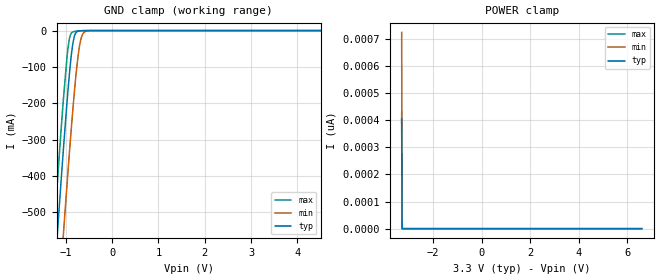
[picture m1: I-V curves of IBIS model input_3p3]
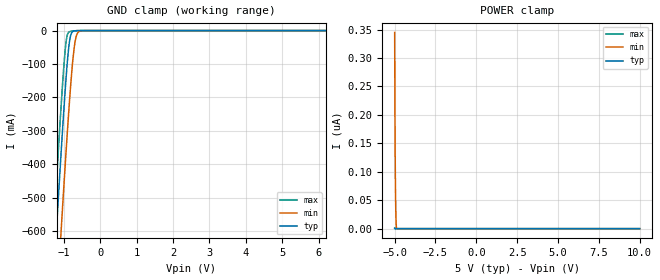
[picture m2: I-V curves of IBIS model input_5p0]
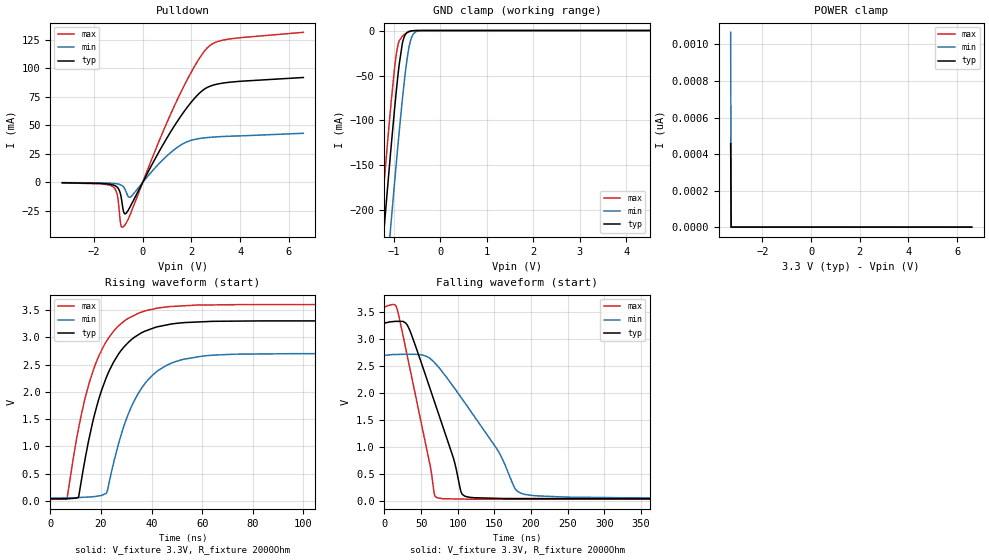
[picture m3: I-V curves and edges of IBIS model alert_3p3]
| Texas Instruments Incorporated
| INA233 High-Side or Low-Side Measurement,
| Bi-Directional Current and Power Monitor with I2C/SMBus/PMBus Compatible Interface
| Marketing part#   Digital Voltage Range   Package-type   #pins
| INA233   2.7V - 5.5V   DGS   10
[IBIS Ver]   4.1
[File name]   ina233.ibs
[Date]   04/25/2017
[File Rev]   1.0
[Source]
| Texas Instruments Incorporated.
| Analog-elab Design Center, HPA
| 12500 TI Blvd
| Dallas, TX -75243
| e-mail: elab_scm_ibis@list.ti.com
[Notes]   Revision History:
| Rev 1.0: 04/25/2017
| - Initial version of the model
| - SDA pin IBIS modeling is done for both
| - Model generated from simulations in SPECTRE
| - Model matched to SPICE simulation
| - C_comp although listed in numerical order of value are
|   obtained from varying PVT conditions. For PVT conditions for
|   each specific value refer the buffer description under
|   respective [Model]. IBIS model user is responsible for using
|   appropriate C_comp to simulate for Signal Integrity.
[Disclaimer]
| This model is designed as an aid for customers of Texas Instruments.
| TI and its licensors and suppliers make no warranties, either expressed
| or implied, with respect to this  model, including the warranties of
| merchantability or fitness for a particular purpose. The model is
| provided solely on an "as is" basis. The entire risk as to its quality
| and performance is with the customer.
[Copyright]
| (C) Copyright 2017 Texas Instruments Incorporated. All rights reserved.
|   INA233
[Component]   INA233
[Manufacturer]  TI
[Package]   |10 VSSOP   -  DGS package
|   typ   min   max
R_pkg   0   0   0
L_pkg   0   0   0
C_pkg   0   0   0
[Pin]  signal_name model_name   R_pin   L_pin   C_pin
1   A1   input   0.05873  1.44199nH  0.22518pF
2   A0   input   0.05490  1.37094nH  0.25227pF
3   Alert   alert   0.05487  1.36860nH  0.25269pF
4   SDA   sda   0.05819  1.42119nH  0.25533pF
5   SCL   scl   0.05921  1.44928nH  0.22479pF
6   VS   power   0.07038  1.61690nH  0.23536pF
7   GND   gnd   0.06315  1.49060nH  0.26023pF
8   VBUS   nc   0.06204  1.47113nH  0.26021pF
9   IN-   nc   0.05785  1.40761nH  0.25629pF
10   IN+   nc   0.07411  1.67461nH  0.23869pF
|   Model Selectors
[Model Selector] input
input_3p3   3.3V  digital Input
input_5p0   5.0V  digital Input
[Model Selector] scl
scl_3p3   3.3V  digital Input
scl_5p0   5.0V  digital Input
[Model Selector] alert
alert_3p3   3.3V  digital Open_drain
alert_5p0   5.0V  digital Open_drain
[Model Selector] sda
sda_3p3   3.3V  digital I/O_Open_drain
sda_5p0   5.0V  digital I/O_Open_drain
sda_hs_3p3   3.3V  digital I/O_Open_drain
sda_hs_5p0   5.0V  digital I/O_Open_drain
| Models and submodels in the file (10): input_3p3 (Input), input_5p0 (Input), alert_3p3 (Open_drain), alert_5p0 (Open_drain), scl_3p3 (Input), scl_5p0 (Input), sda_hs_3p3 (I/O_open_drain), sda_hs_5p0 (I/O_open_drain), sda_3p3 (I/O_open_drain), sda_5p0 (I/O_open_drain)
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|   input_3p3
[Model]   input_3p3
Model_type   Input
Vinl = 0.4
Vinh = 2.31
|   typ   min   max
C_comp   6.158E-13   5.919E-13   6.357E-13
| Where Nom  PVT is Nominal Process, 3.3V, 25C
|   Fast PVT is Strong Process,  3.6V, -40C
|   Slow PVT is Weak Process,   2.7V, 125C
[Voltage Range]   3.3   2.7   3.6
[Temperature Range]   25   125   -40
[Power Clamp Reference]   3.3   2.7   3.6
[GND Clamp Reference]   0   0   0
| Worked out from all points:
|   GND clamp passes 1 mA (typ) near -0.71 V on its own axis
[GND Clamp]
|   Voltage   I(typ)   I(min)   I(max)
-3.3V     -4.686A    -4.907A    -4.556A
-1.251V   -685.9mA   -923.4mA   -543.4mA
-1.181V   -558mA     -795.1mA   -415.7mA
-1.053V   -328.1mA   -561.6mA   -190.2mA
-953.7mV  -165.6mA   -388.9mA   -49.35mA
-904.2mV  -95.52mA   -306.4mA   -13.32mA
-844.8mV  -33.22mA   -212.7mA   -3.47mA
-765.6mV  -3.856mA   -104mA     -1.449mA
-696.3mV  -740.9uA   -37.2mA    -647.4uA
-636.9mV  -214.4uA   -10.28mA   -278.8uA
-547.8mV  -30.3uA    -1.138mA   -47.56uA
6.6V      0A         0A         0A
[POWER Clamp]
|   Voltage   I(typ)   I(min)   I(max)
-3.3V     403.7pA    722.8pA    427pA
-3.28V    0A         0A         0A
-3.27V    0A         0A         0A
6.6V      0A         0A         0A
|   input_5p0
[Model]   input_5p0
Model_type   Input
Vinl = 0.4
Vinh = 3.5
|   typ   min   max
C_comp   6.144E-13   5.916E-13   6.351E-13
| Where Nom  PVT is Nominal Process, 5V, 25C
|   Fast PVT is Strong Process,  5.5V, -40C
|   Slow PVT is Weak Process,   4.5V, 125C
[Voltage Range]   5   4.5   5.5
[Temperature Range]   25   125   -40
[Power Clamp Reference]   5   4.5   5.5
[GND Clamp Reference]   0   0   0
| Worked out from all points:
|   GND clamp passes 1 mA (typ) near -0.71 V on its own axis
[GND Clamp]
|   Voltage   I(typ)   I(min)   I(max)
-5V       -8.058A    -8.271A    -7.934A
-1.43V    -1.024A    -1.261A    -882.3mA
-1.25V    -684.6mA   -922.1mA   -542.1mA
-1.235V   -656.8mA   -894.2mA   -514.2mA
-1.175V   -546.3mA   -783.3mA   -404mA
-1.085V   -384.5mA   -619.4mA   -244.5mA
-950mV    -160mA     -382.6mA   -45.51mA
-905mV    -96.55mA   -307.7mA   -13.63mA
-830mV    -23.26mA   -190.7mA   -2.862mA
-695mV    -720.9uA   -36.31mA   -637uA
-515mV    -13.73uA   -522.2uA   -21.3uA
10V       0A         0A         0A
[POWER Clamp]
|   Voltage   I(typ)   I(min)   I(max)
-5V       635.3pA    344.9nA    1.296nA
-4.985V   317.6pA    207.1nA    647.8pA
-4.97V    0A         128.5nA    0A
-4.955V   0A         77.65nA    0A
-4.94V    0A         44.8nA     0A
-4.925V   0A         23.57nA    0A
-4.91V    0A         9.855nA    0A
-4.895V   0A         994.4pA    0A
-4.865V   0A         0A         0A
10V       0A         0A         0A
|   alert_3p3
[Model]   alert_3p3
Model_type   Open_drain
Polarity   Non-Inverting
Vmeas = 1.65
Vref = 3.3
Cref = 2pF
Rref = 2000
|   typ   min   max
C_comp   1.362E-12   1.340E-12   1.377E-12
| C_comp_Pull_Down   1.226E-12   1.207E-12   1.271E-12
| Where Nom  PVT is Nominal Process, 3.3V, 25C
|   Fast PVT is Strong Process,  3.6V, -40C
|   Slow PVT is Weak Process,   2.7V, 125C
[Voltage Range]   3.3   2.7   3.6
[Temperature Range]   25   125   -40
[Pullup Reference]   3.3   2.7   3.6
[Pulldown Reference]   0   -0   0
[Power Clamp Reference]   3.3   2.7   3.6
[GND Clamp Reference]   0   0   0
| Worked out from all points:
|   slope of the pulldown table from 0 to 0.495 V, typ, clamps not added: 24.6 ohm
|   GND clamp passes 1 mA (typ) near -0.67 V on its own axis
|   falling waveform, V_fixture 3.3V, R_fixture 2000Ohm: 20-80 % time 48.2ns typ, 76ns min, 32.9ns max; typ from 3.3 V to 0.038 V
|   rising waveform, V_fixture 3.3V, R_fixture 2000Ohm: 20-80 % time 12.9ns typ, 13.3ns min, 12.7ns max; typ from 0.038 V to 3.3 V
[Pulldown]
|   Voltage   I(typ)   I(min)   I(max)
-3.3V     -289.2uA   -143.4uA   -364.9uA
-1.211V   -2.249mA   -851.9uA   -3.91mA
-1.043V   -4.246mA   -1.29mA    -10.92mA
-943.8mV  -7.802mA   -1.798mA   -29.35mA
-884.4mV  -12.88mA   -2.307mA   -38.4mA
-815.1mV  -22.41mA   -3.305mA   -39.12mA
-735.9mV  -27.53mA   -5.582mA   -37.44mA
-498.3mV  -20.66mA   -12.76mA   -27.41mA
1.264V    48.27mA    28.21mA    65.31mA
2.63V     83.03mA    39.29mA    117.5mA
3.482V    87.62mA    40.44mA    125.5mA
6.6V      91.99mA    43.09mA    131.6mA
[GND Clamp]
|   Voltage   I(typ)   I(min)   I(max)
-3.3V     -1.581A    -1.661A    -1.533A
-1.33V    -296.5mA   -381.4mA   -245.5mA
-1.211V   -222.5mA   -307.3mA   -171.5mA
-1.073V   -138.7mA   -222.6mA   -89.06mA
-983.4mV  -87.83mA   -169.6mA   -42.34mA
-933.9mV  -61.66mA   -141.1mA   -22.64mA
-884.4mV  -38.28mA   -113.4mA   -11.66mA
-815.1mV  -14.34mA   -76.79mA   -6.359mA
-676.5mV  -1.172mA   -19.9mA    -1.628mA
-577.5mV  -162.7uA   -3.87mA    -278.3uA
-419.1mV  -2.695uA   -102.7uA   -3.38uA
6.6V      0A         0A         0A
[POWER Clamp]
|   Voltage   I(typ)   I(min)   I(max)
-3.3V     456.9pA    1.067nA    491.6pA
-3.28V    0A         0A         0A
-3.27V    0A         0A         0A
6.6V      0A         0A         0A
[Ramp]
R_load = 2000
|   typ   min   max
dV/dt_r   1.95743/1.28876e-08   1.58891/1.33026e-08   2.1419/1.27257e-08
dV/dt_f   1.95743/4.81415e-08   1.58891/7.59786e-08   2.1419/3.29056e-08
[Falling Waveform]
V_fixture = 3.3V
V_fixture_min = 2.7V
V_fixture_max = 3.6V
R_fixture = 2000Ohm
C_fixture = 0F
|   Time   V(typ)   V(min)   V(max)
0s        3.3V       2.7V       3.6V
18.03ns   3.322V     2.711V     3.515V
33.33ns   3.195V     2.713V     2.541V
62.38ns   2.07V      2.633V     649.6mV
67.88ns   1.849V     2.566V     140mV
70.98ns   1.724V     2.52V      64.27mV
94.47ns   772.9mV    2.106V     37.86mV
106.2ns   122.8mV    1.883V     34.96mV
185.3ns   44.62mV    147.8mV    32.77mV
500ns     37.62mV    51.82mV    30.17mV
[Rising Waveform]
V_fixture = 3.3V
V_fixture_min = 2.7V
V_fixture_max = 3.6V
R_fixture = 2000Ohm
C_fixture = 0F
|   Time   V(typ)   V(min)   V(max)
0s        37.62mV    51.82mV    30.17mV
6.604ns   41.41mV    56.46mV    37.55mV
11.12ns   64.81mV    62.75mV    1.316V
16.71ns   1.435V     77.27mV    2.353V
22.15ns   2.263V     141.9mV    2.923V
30.71ns   2.899V     1.58V      3.344V
36.29ns   3.087V     2.082V     3.465V
42.26ns   3.191V     2.377V     3.532V
73.19ns   3.295V     2.69V      3.597V
500ns     3.3V       2.7V       3.6V
